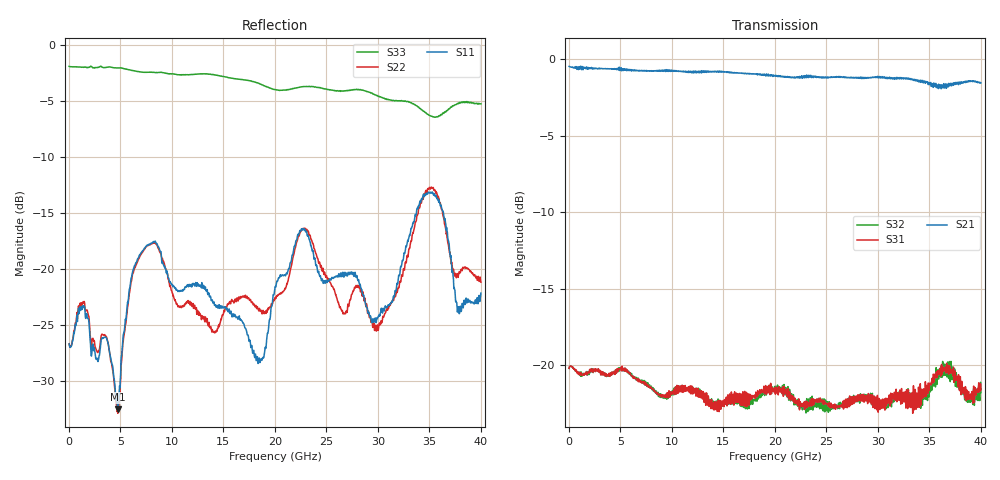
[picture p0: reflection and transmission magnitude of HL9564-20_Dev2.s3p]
! 10/7/2020 12:26:43 PM
! H:\PRODUCTION_DATA\TEMP_S3P.S3P
! CHANNEL.1
! TR.MEASUREMENT
! CORRECTED.DATA
# GHZ S RI R 50.0
! FREQ.GHZ  S11RE  S11IM  S12RE  S12IM  S13RE  S13IM
!  S21RE  S21IM  S22RE  S22IM  S23RE  S23IM
!  S31RE  S31IM  S32RE  S32IM  S33RE  S33IM
!; PortSelection: Port_123
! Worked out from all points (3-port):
!   1143 points, 35 MHz to 40.01 GHz, reference 50 ohm
!   strongest paths, dB at 35 MHz, 10.01 GHz, 20.02 GHz, 30.03 GHz, 40.01 GHz:
!     S21: -0.5, -0.8, -1.1, -1.2, -1.5
!     S31: -20.2, -21.9, -21.7, -23.1, -21.6
!     S32: -20.2, -21.9, -21.7, -22.7, -21.8
!   lowest |S11| = -32.6 dB at 4.76 GHz (marker M1), VSWR 1.05, Z = 48.1 - j1.37 ohm
!   |S11| at or under -10 dB: start of sweep to end of sweep
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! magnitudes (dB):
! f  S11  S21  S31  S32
! 35 MHz  -26.7  -0.5  -20.2  -20.2
! 4.76 GHz  -32.6  -0.7  -20.4  -20.4
! 7.63 GHz  -17.8  -0.8  -21.3  -21.2
! 18.41 GHz  -28.3  -1.0  -21.9  -22.2
! 20.02 GHz  -21.7  -1.1  -21.7  -21.7
! 22.93 GHz  -16.5  -1.1  -22.6  -22.5
! 29.89 GHz  -24.5  -1.2  -22.9  -22.7
! 35.1 GHz  -13.2  -1.5  -21.2  -21.7
! 37.77 GHz  -23.5  -1.5  -21.3  -20.8
! 40.01 GHz  -22.2  -1.5  -21.6  -21.8
